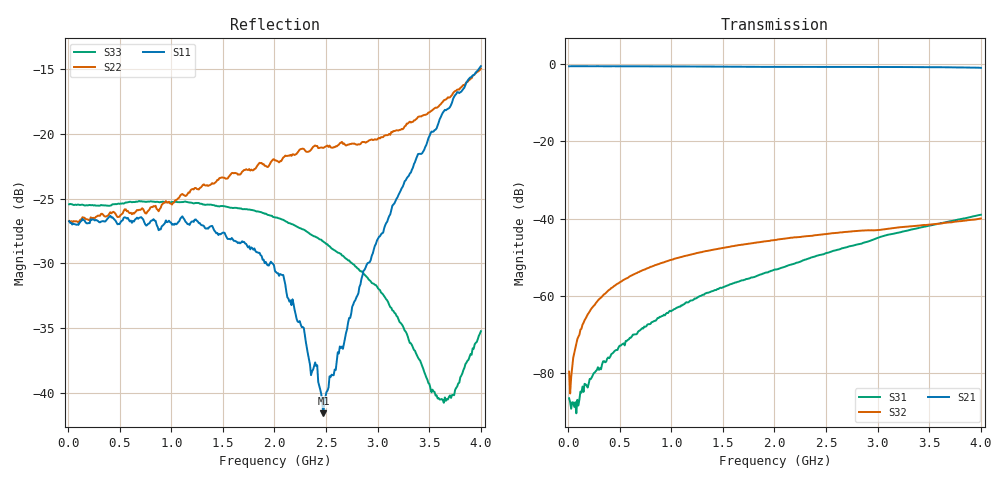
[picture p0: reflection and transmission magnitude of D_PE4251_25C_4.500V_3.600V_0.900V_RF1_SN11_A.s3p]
! Device ID: PE4251_SoldCshunt_081809
! Dir: c:\Test Bench Repositories\Bench_Software_CVI_Version_8\trunk\PSC 4Port_VNA Bench\datalog\4250\TEST\PE4251_SoldCshunt_081809\25C\4p500000\RF1
! Serial: 11
! Insertion: A
! Temp: 25C
! VDD: 4.500
! Control_Hi: 80.000
! Control_Lo: 20.000
! Logic State: RF1
! Port 1: RFC
! Port 2: RF1
! Port 3: RF2
! V1 = 0.90
! V2 = 3.60
! V3 = 0.90
! IDD: 5.849970e-05
! FILE NAME
! DATE 08/18/09  20:13
! CORRECTED  DATA
#  Hz  S  RI  R  50.00
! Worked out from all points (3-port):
!   401 points, 10 MHz to 4 GHz, reference 50 ohm
!   strongest paths, dB at 10 MHz, 1.008 GHz, 2.005 GHz, 3.002 GHz, 4 GHz:
!     S21: -0.6, -0.6, -0.7, -0.7, -1.0
!     S32: -79.6, -50.6, -45.5, -43.0, -39.9
!     S31: -86.4, -63.8, -53.1, -44.9, -39.0
!   lowest |S11| = -41.6 dB at 2.474 GHz (marker M1), VSWR 1.02, Z = 50 - j0.831 ohm
!   |S11| at or under -10 dB: start of sweep to end of sweep
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1e7  0.046 2.1e-05  0.9377 -0.00322  1.04e-05 -7.81e-05
     0.9375 -0.00458  0.0461 -1.8e-05  2.48e-05 3.56e-05
     1.32e-05 -4.58e-05  0.000104 1.76e-05  0.0534 -0.000519
9.9775e7  0.0445 -0.000764  0.9394 -0.0342  2.69e-05 -4.05e-05
          0.9387 -0.0346  0.0455 -0.000701  3.73e-05 0.000295
          1.08e-05 -3.68e-05  4.26e-05 0.000295  0.0533 -0.000506
1.8955e8  0.0451 0.000129  0.9363 -0.0642  -1.04e-05 -7.73e-05
          0.9359 -0.0645  0.0467 -0.000241  6.52e-05 0.000571
          -3.12e-06 -6.54e-05  5.5e-05 0.000575  0.0529 -0.00117
4.98775e8  0.0446 -0.00448  0.9212 -0.1653  -0.000147 -0.000173
           0.9209 -0.1647  0.0478 -0.0036  0.00015 0.00149
           -0.000149 -0.000172  0.000147 0.00149  0.0534 -0.0046
1.137175e9  0.0429 -0.0159  0.8583 -0.3623  -0.000761 -0.000253
            0.8585 -0.3614  0.0549 -0.0173  0.000578 0.00325
            -0.000771 -0.000266  0.000579 0.00326  0.0544 -0.00652
2.005e9  0.0265 -0.0129  0.7154 -0.5805  -0.00219 -0.000162
         0.7155 -0.5803  0.0688 -0.0387  0.0011 0.00518
         -0.0022 -0.000167  0.00111 0.0052  0.0474 -0.00409
2.473825e9  -0.000284 -0.00832  0.6213 -0.6765  -0.00348 -0.000153
            0.6186 -0.6749  0.0631 -0.0617  0.00123 0.00613
            -0.00346 -0.000156  0.00123 0.00614  0.0384 -6.94e-05
2.872825e9  -0.0197 -0.0225  0.5275 -0.7513  -0.00495 2.42e-05
            0.5293 -0.7493  0.0426 -0.0827  0.00128 0.00691
            -0.00494 1.31e-05  0.0013 0.00693  0.0284 0.00269
3.62095e9  -0.0989 -0.0655  0.3121 -0.8536  -0.0086 0.00171
           0.3134 -0.8548  -0.0463 -0.1234  0.000324 0.00871
           -0.00863 0.0017  0.000326 0.00869  0.00225 0.00918
4e9  -0.1643 -0.0799  0.1786 -0.8796  -0.0108 0.00311
     0.1785 -0.8761  -0.1262 -0.1268  -0.000349 0.01
     -0.0108 0.0031  -0.000377 0.0101  -0.0136 0.0106
